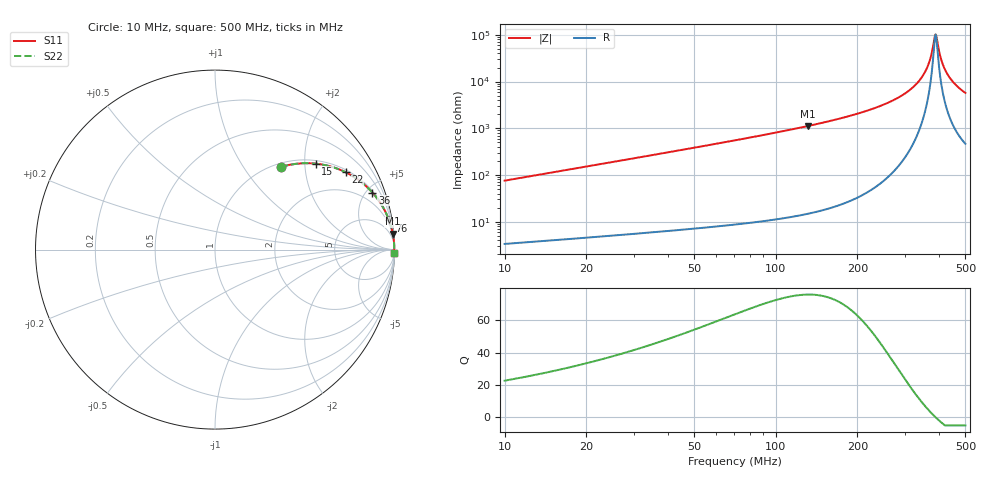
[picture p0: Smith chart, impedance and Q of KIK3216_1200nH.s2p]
!version-2
!date-01.2022
!Series
# MHz S RI R 50
!Freq ReS11 ImS11 ReS21 ImS21 ReS12 ImS12 ReS22 ImS22
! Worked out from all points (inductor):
!   491 points, 10 MHz to 500 MHz, reference 50 ohm
!   read as one part in series: L = 1.2 uH near 12 MHz
!   highest Q = 75.8 at 131 MHz (marker M1), where L = 1.35 uH
!   self-resonance near 388 MHz
!   S11 on the Smith chart (normalised r, x): 10 MHz: 1.07, +1.51; 15 MHz: 1.08, +2.27; 22 MHz: 1.09, +3.33; 36 MHz: 1.12, +5.48; 76 MHz: 1, +12; 500 MHz: open
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10  0.3688 0.4609  0.6312 -0.4609  0.6312 -0.4609  0.3688 0.4609
15  0.5602 0.4791  0.4398 -0.4791  0.4398 -0.4791  0.5602 0.4791
22  0.7291 0.4304  0.2709 -0.4304  0.2709 -0.4304  0.7291 0.4304
36  0.877 0.3176  0.123 -0.3176  0.123 -0.3176  0.877 0.3176
76  0.9703 0.1624  0.0297 -0.1624  0.0297 -0.1624  0.9703 0.1624
92  0.98 0.1331  0.02 -0.1331  0.02 -0.1331  0.98 0.1331
131  0.9909 0.0888  0.00914 -0.0888  0.00914 -0.0888  0.9909 0.0888
174  0.9955 0.0606  0.00455 -0.0606  0.00455 -0.0606  0.9955 0.0606
255  0.9984 0.0295  0.0016 -0.0295  0.0016 -0.0295  0.9984 0.0295
303  0.9989 0.0171  0.00106 -0.0171  0.00106 -0.0171  0.9989 0.0171
337  0.9991 0.0097  0.000931 -0.0097  0.000931 -0.0097  0.9991 0.0097
353  0.9991 0.00652  0.000918 -0.00652  0.000918 -0.00652  0.9991 0.00652
366  0.9991 0.00405  0.000927 -0.00405  0.000927 -0.00405  0.9991 0.00405
375  0.9991 0.00239  0.000942 -0.00239  0.000942 -0.00239  0.9991 0.00239
385  0.999 0.000597  0.000967 -0.000597  0.000967 -0.000597  0.999 0.000597
388  0.999 6.85e-05  0.000976 -6.85e-05  0.000976 -6.85e-05  0.999 6.85e-05
391  0.999 -0.000456  0.000986 0.000456  0.000986 0.000456  0.999 -0.000456
399  0.999 -0.00184  0.00102 0.00184  0.00102 0.00184  0.999 -0.00184
405  0.999 -0.00285  0.00104 0.00285  0.00104 0.00285  0.999 -0.00285
419  0.9989 -0.00517  0.00111 0.00517  0.00111 0.00517  0.9989 -0.00517
451  0.9987 -0.0102  0.00131 0.0102  0.00131 0.0102  0.9987 -0.0102
500  0.9983 -0.0174  0.00172 0.0174  0.00172 0.0174  0.9983 -0.0174
